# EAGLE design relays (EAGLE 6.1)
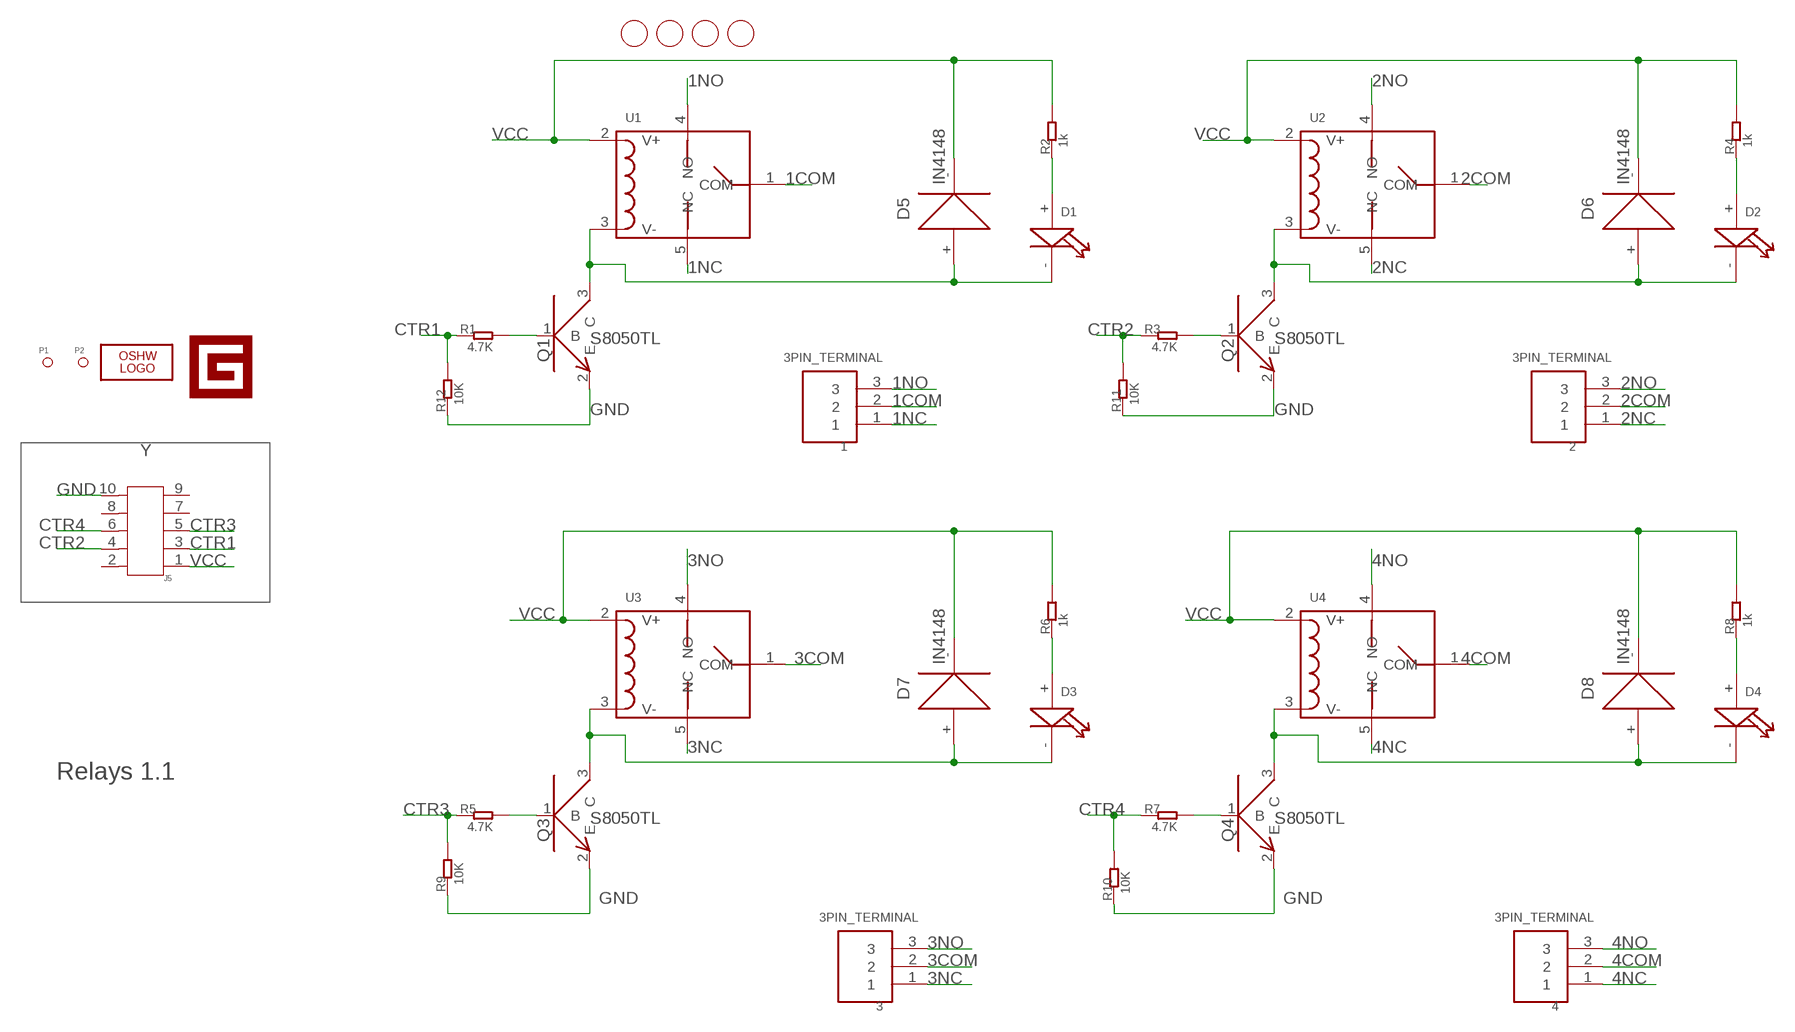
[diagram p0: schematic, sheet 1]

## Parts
1  3PIN_TERMINAL  [3PIN_TERMINAL]
2  3PIN_TERMINAL  [3PIN_TERMINAL]
3  3PIN_TERMINAL  [3PIN_TERMINAL]
4  3PIN_TERMINAL  [3PIN_TERMINAL]
D1  LED0805  [LED0805]
D2  LED0805  [LED0805]
D3  LED0805  [LED0805]
D4  LED0805  [LED0805]
D5  IN4148  DIODE1206  [DIODE1206]
D6  IN4148  DIODE1206  [DIODE1206]
D7  IN4148  DIODE1206  [DIODE1206]
D8  IN4148  DIODE1206  [DIODE1206]
J5  HEADER-SHF-105-01-L-D-SM  [SHF-105-01-L-D-SM]
LOGO1  LOGO-OSHW-FILLX0150-NT  [OSHW_FILLX150_NOTEXT]
P1  PAD-MARK  [ROUND-MARK-0.635]
P2  PAD-MARK  [ROUND-MARK-0.635]
Q1  NPN_9013  [SOT23]
Q2  NPN_9013  [SOT23]
Q3  NPN_9013  [SOT23]
Q4  NPN_9013  [SOT23]
R1  4.7K  R0603  [0603]
R2  1k  R0603  [0603]
R3  4.7K  R0603  [0603]
R4  1k  R0603  [0603]
R5  4.7K  R0603  [0603]
R6  1k  R0603  [0603]
R7  4.7K  R0603  [0603]
R8  1k  R0603  [0603]
R9  10K  R0603  [0603]
R10  10K  R0603  [0603]
R11  10K  R0603  [0603]
R12  10K  R0603  [0603]
U1  RELAY  [5P-LEADED-17X21.6]
U2  RELAY  [5P-LEADED-17X21.6]
U3  RELAY  [5P-LEADED-17X21.6]
U4  RELAY  [5P-LEADED-17X21.6]
U$1  PAD-HOLE'3.2/7.0'  [HOLE-D-3.2/7.0]
U$2  PAD-HOLE'3.2/7.0'  [HOLE-D-3.2/7.0]
U$3  PAD-HOLE'3.2/7.0'  [HOLE-D-3.2/7.0]
U$4  PAD-HOLE'3.2/7.0'  [HOLE-D-3.2/7.0]
U$5  LOGO-GADGETEER-NORMAL  [GADGETEER-SILK]

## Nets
1COM: 1.2 U1.1(COM)
1NC: 1.1 U1.5(NC)
1NO: 1.3 U1.4(NO)
2COM: 2.2 U2.1(COM)
2NC: 2.1 U2.5(NC)
2NO: 2.3 U2.4(NO)
3COM: 3.2 U3.1(COM)
3NC: 3.1 U3.5(NC)
3NO: 3.3 U3.4(NO)
4COM: 4.2 U4.1(COM)
4NC: 4.1 U4.5(NC)
4NO: 4.3 U4.4(NO)
CTR1: J5.3 R1.1 R12.2
CTR2: J5.4 R3.1 R11.2
CTR3: J5.5 R5.1 R9.2
CTR4: J5.6 R7.1 R10.2
GND: J5.10 Q1.2(E) Q2.2(E) Q3.2(E) Q4.2(E) R9.1 R10.1 R11.1 R12.1
N$2: Q1.1(B) R1.2
N$3: D2.+ R4.1
N$4: Q2.1(B) R3.2
N$5: D3.+ R6.1
N$6: D3.- D7.+ Q3.3(C) U3.3(V-)
N$7: D4.+ R8.1
N$8: Q4.1(B) R7.2
N$9: D2.- D6.+ Q2.3(C) U2.3(V-)
N$10: Q3.1(B) R5.2
N$12: D1.- D5.+ Q1.3(C) U1.3(V-)
N$13: D1.+ R2.1
N$18: D4.- D8.+ Q4.3(C) U4.3(V-)
VCC: D5.- D6.- D7.- D8.- J5.1 R2.2 R4.2 R6.2 R8.2 U1.2(V+) U2.2(V+) U3.2(V+) U4.2(V+)
Unconnected: J5.2 J5.7 J5.8 J5.9

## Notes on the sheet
- S8050TL | S8050TL
- Y
- Relays 1.1
- S8050TL | S8050TL

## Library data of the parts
1-4 = Seeed:3PIN_TERMINAL
D1-D4 = CPT_SMD:LED0805
D5-D8 = CPT_SMD:DIODE
J5 = Connector:HEADER-SHF-105-01-L-D-SM
LOGO1 = Logo:LOGO-OSHW-FILL
P1 P2 = Discreter:PAD-MARK
Q1-Q4 = CPT_SMD:NPN_9013
R1-R12 = CPT_SMD:R0603
U1-U4 = Discreter:RELAY
U$1-U$4 = Discreter:PAD-HOLE
U$5 = Logo:LOGO-GADGETEER

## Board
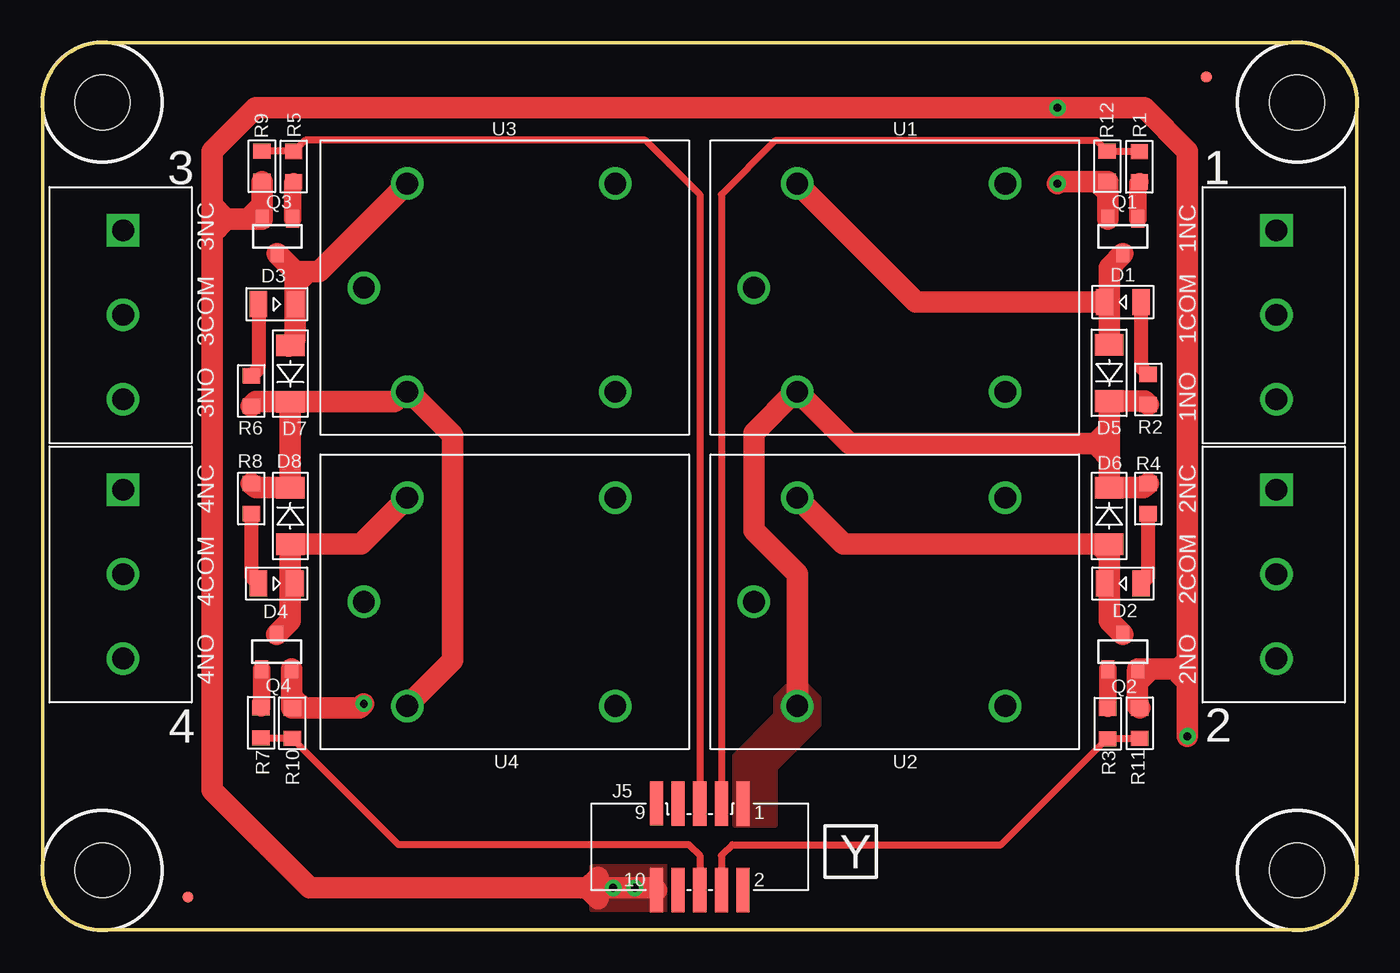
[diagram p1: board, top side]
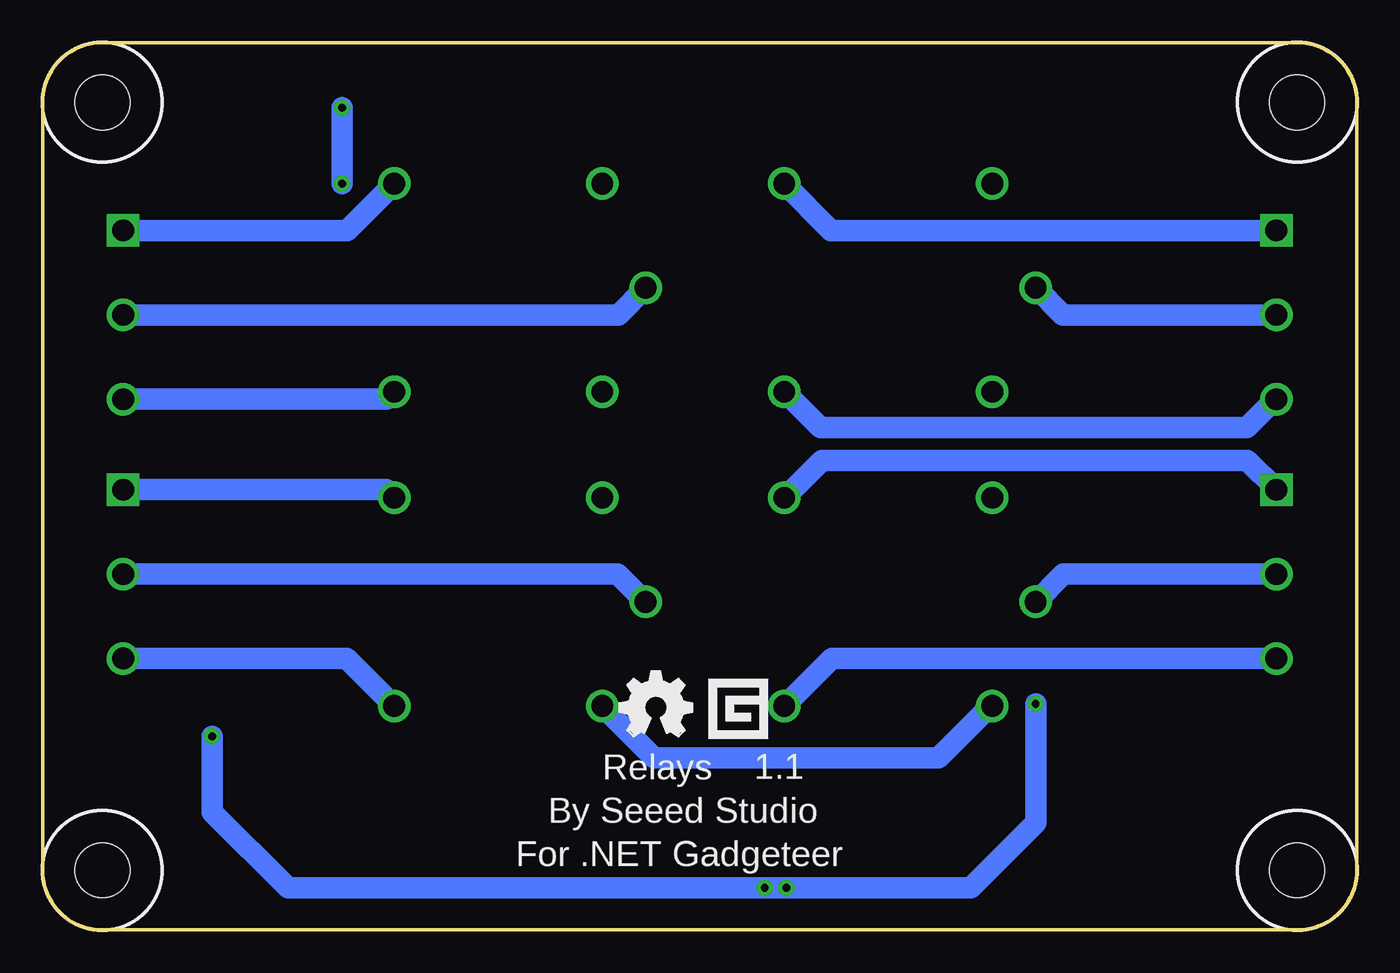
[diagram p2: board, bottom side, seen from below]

Size 77 x 52 mm. Coordinates in mm from the lower left corner, seen from the top.
Outline: 0,48.5 arc-90 3.5,52 73.5,52 arc-90 77,48.5 77,3.5 arc-90 73.5,0 3.5,0 arc-90 0,3.5 0,48.5
Copper layers (1*16): Top 0.035mm / dielectric 1.5mm / Bottom 0.035mm
Design rules: minimum track width 7mil, minimum drill 12mil, track to track 8mil, track to pad 8mil, pad to pad 8mil, via to via 8mil, smd to smd 8mil, copper to edge 20mil, drill to drill 8mil, minimum pad ring 10mil, minimum via ring 8mil, stop-mask expansion 4mil, vias tented up to drill 25mil, thermal gap 10mil

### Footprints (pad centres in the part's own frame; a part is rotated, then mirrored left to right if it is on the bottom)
3PIN_TERMINAL = drill 1.27 pad 1.778 square: 1 0,0 | drill 1.27 pad 1.778: 2 0,4.95; 3 0,9.893
LED0805 = smd 1.016 x 1.524: + -1.077,0; - 1.077,0
DIODE1206 = smd 1.27 x 1.651: + -1.651,0; - 1.651,0
SHF-105-01-L-D-SM = smd 0.762 x 2.6: 1 -2.54,-2.54; 2 -2.54,2.54; 3 -1.27,-2.54; 4 -1.27,2.54; 5 0,-2.54; 6 0,2.54; 7 1.27,-2.54; 8 1.27,2.54; 9 2.54,-2.546; 10 2.54,2.54
ROUND-MARK-0.635 = smd 0.635 x 0.635: P$1 0,0
SOT23 = smd 0.762 x 1.016: 1 -0.889,-1.016; 2 0.889,-1.016; 3 0,1.016
0603 = smd 0.889 x 1.016: 1 -0.889,0; 2 0.889,0
5P-LEADED-17X21.6 = drill 1.27: 1 -2.54,-6.096; 2 0,-12.192; 3 0,0; 4 12.192,-12.192; 5 12.192,0
HOLE-D-3.2/7.0 = hole 3.2: 0,0

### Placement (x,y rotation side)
1  72.28,41 180 top
2  72.28,25.81 180 top
3  4.72,41 180 top
4  4.72,25.81 180 top
D1  63.29,36.8 180 top
D2  63.29,20.3 180 top
D3  13.72,36.67 0 top
D4  13.71,20.3 0 top
D5  62.49,32.65 270 top
D6  62.49,24.27 90 top
D7  14.51,32.61 270 top
D8  14.51,24.27 90 top
J5  38.5,4.88 180 top
LOGO1  43.2,11.36 0 bottom
P1  8.51,1.94 0 top
P2  68.18,50 0 top
Q1  63.29,40.65 180 top
Q2  63.29,16.31 0 top
Q3  13.75,40.65 180 top
Q4  13.71,16.31 0 top
R1  64.26,44.73 270 top
R2  64.77,31.68 270 top
R3  62.4,12.09 90 top
R4  64.77,25.28 90 top
R5  14.71,44.74 270 top
R6  12.23,31.59 270 top
R7  12.8,12.14 90 top
R8  12.23,25.28 90 top
R9  12.85,44.76 90 top
R10  14.62,12.12 270 top
R11  64.28,12.12 270 top
R12  62.38,44.76 90 top
U1  44.22,43.74 0 top
U2  44.22,25.32 0 top
U3  21.36,43.74 0 top
U4  21.36,25.32 0 top
U$1  73.5,48.5 0 top
U$2  73.5,3.5 0 top
U$3  3.5,48.5 0 top
U$4  3.5,3.5 0 top
U$5  35.83,13.39 0 bottom

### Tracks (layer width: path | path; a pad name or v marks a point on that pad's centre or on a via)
1COM
  Bottom 1.27: 1.2 43.27,36.05 U1.1
1NC
  Bottom 1.27: 1.1 59.15,41 U1.5
1NO
  Bottom 1.27: 1.3 56.85,31.1 U1.4
2COM
  Bottom 1.27: 2.2 43.3,20.86 U2.1
2NC
  Bottom 1.27: 2.1 56.89,25.81 U2.5
2NO
  Bottom 1.27: 2.3 59.19,15.91 U2.4
3COM
  Bottom 1.27: 3.2 17.22,36.05 U3.1
3NC
  Bottom 1.27: 3.1 30.8,41 U3.5
3NO
  Bottom 1.27: 3.3 4.78,31.1 6.44,29.44 31.44,29.44 U3.4
4COM
  Bottom 1.27: 4.2 17.19,20.86 U4.1
4NC
  Bottom 1.27: 4.1 4.72,25.83 6.41,27.52 31.35,27.52 U4.5
4NO
  Bottom 1.27: 4.3 30.77,15.91 U4.4
CTR1
  Top 0.406: J5.3 39.77,43.11 42.95,46.28 61.74,46.28 R12.2 64.23,45.64 R1.1
CTR2
  Top 0.178: R3.1 62.48,11.2 62.5,11.23
  Top 0.406: J5.4 39.77,4.37 40.41,5 56.15,5 62.38,11.23 62.5,11.23 R11.2
CTR3
  Top 0.406: J5.5 38.5,43.11 35.33,46.28 15.39,46.28 14.74,45.63 R5.1 12.86,45.63 R9.2
CTR4
  Top 0.406: J5.6 38.5,4.37 37.87,5 20.85,5 R10.2 12.82,11.23 R7.1
GND  (via drill 0.46 pad 0.97)
  Top 1.27: J5.10 35.83,2.46 v33.42,2.46 31.9,2.46 | 9.93,40.82 9.93,8.18 15.64,2.46 31.9,2.46 | 9.93,40.82 9.93,41.84 | 9.93,41.84 9.93,42.47 | 9.93,42.47 9.93,45.64 12.46,48.19 v59.45,48.19 64.53,48.19 67.08,45.64 67.08,15.8 | 67.08,14.53 67.08,15.8 | v67.08,11.36 67.08,14.53 | 66.57,15.29 64.92,15.29 | 64.92,15.29 64.28,15.29 | 64.28,15.29 Q2.2 | 67.08,15.8 66.57,15.29 | 66.57,15.29 66.57,15.04 67.08,14.53 | 10.73,41.67 10.09,41.67 9.93,41.84 | 10.75,41.67 12.12,41.67 | 12.12,41.67 Q3.2 12.86,43.85 R9.1 | 10.75,41.67 10.73,41.67 | 9.93,42.47 10.73,41.67 | 10.75,41.67 10.75,41.65 9.93,40.82 | 31.9,2.46 32.53,3.1 | 31.9,2.46 32.53,1.83 | 12.12,41.67 12.12,41.75 12.85,42.47 | Q1.2 62.4,43.84 | 62.4,43.84 R12.1 | 62.4,43.84 61.77,43.84 | v59.45,43.74 59.56,43.84 61.7,43.84 61.77,43.84 | 64.28,15.29 64.15,15.16 64.15,13.13 R11.1 | 64.92,15.29 64.28,14.66 | Q4.2 14.6,13.67 | 14.6,13.67 14.6,13.03 R10.1 15.26,13.01 | 15.26,13.01 18.56,13.01 v18.82,13.26 | 14.6,13.67 15.26,13.01 | 61.77,43.84 62.38,43.23
  Bottom 1.27: v18.82,13.26 18.82,6.27 22.62,2.46 v33.42,2.46 62.63,2.46 67.08,6.91 v67.08,11.36 | v59.45,48.19 v59.45,43.74
  other vias: 34.69,2.46
  pour Top (isolate 0.254, no thermals): 32.15,3.73 36.59,3.73 36.59,1.2 32.15,1.2
N$2
  Top 1.016: Q1.1 64.18,43.77 R1.2 64.28,43.87
N$3
  Top 0.813: R4.1 64.77,20.7 D2.+
N$4
  Top 1.016: Q2.1 R3.2
N$5
  Top 0.813: D3.+ 12.64,32.9 R6.1
N$6
  Top 1.27: 14.8,38.59 14.8,37.82 | 14.8,38.59 Q3.3 | 14.8,38.59 16.2,38.59 U3.3 | D7.+ 14.47,34.22 14.37,34.22 14.8,34.64 D3.- 14.8,37.65 14.8,37.82 | 14.8,37.82 15.39,38.41
N$7
  Top 0.813: R8.1 12.23,20.7 D4.+
N$8
  Top 1.016: Q4.1 12.82,13.06 R7.2
N$9
  Top 0.813: D2.- 62.44,20.3 62.49,20.24 | 60.67,22.62 61.53,22.62 62.63,21.52
  Top 1.27: U2.3 46.92,22.62 60.67,22.62 D6.+ 62.49,20.24 62.49,18.13 Q2.3
N$10
  Top 1.016: Q3.1 14.64,43.78 R5.2
N$12
  Top 0.813: D1.- 62.45,36.8 62.49,36.76
  Top 1.27: D5.+ 62.49,36.76 62.49,38.83 Q1.3 | 62.45,36.8 51.16,36.8 U1.3
N$13
  Top 0.813: D1.+ 64.37,32.97 R2.1
N$18
  Top 0.813: D4.- 14.56,20.3 14.51,20.24
  Top 1.27: U4.3 18.65,22.62 D8.+ 14.51,20.24 14.51,18.13 Q4.3
VCC
  Top 0.813: 62.63,29.77 61.36,28.5 62.63,27.23
  Top 1.27: R4.2 64.52,25.92 D6.- 62.49,28.5 | R2.2 64.77,30.8 64.58,31 D5.- 62.49,28.5 | D7.- 12.48,30.95 R6.2 | D7.- 20.64,30.95 21.36,31.68 U3.2 21.48,31.55 24.03,29 24.03,15.81 U4.2 | R8.2 12.48,25.92 D8.- D7.- | 62.49,28.5 61.36,28.5 47.26,28.5 U1.2 44.09,31.55 41.67,29.14 41.67,23.42 44.22,20.88 U2.2
  Bottom 1.27: U4.2 21.48,13.13 24.53,10.09 41.17,10.09 U2.2
  pour Top (isolate 0.254, no thermals): 40.53,6.15 40.53,10.21 42.95,12.62 42.95,13.63 43.84,14.53 44.59,14.53 45.48,13.63 45.48,11.99 42.95,9.45 42.95,6.15

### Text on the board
tPlace: 3NC | 1NC | 3COM | 1COM | 3NO | 1NO | 4NC | 2NC | 2COM | 4COM | 4NO | 2NO | Y
bPlace: 1.1 | Relays | By Seeed Studio | For .NET Gadgeteer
